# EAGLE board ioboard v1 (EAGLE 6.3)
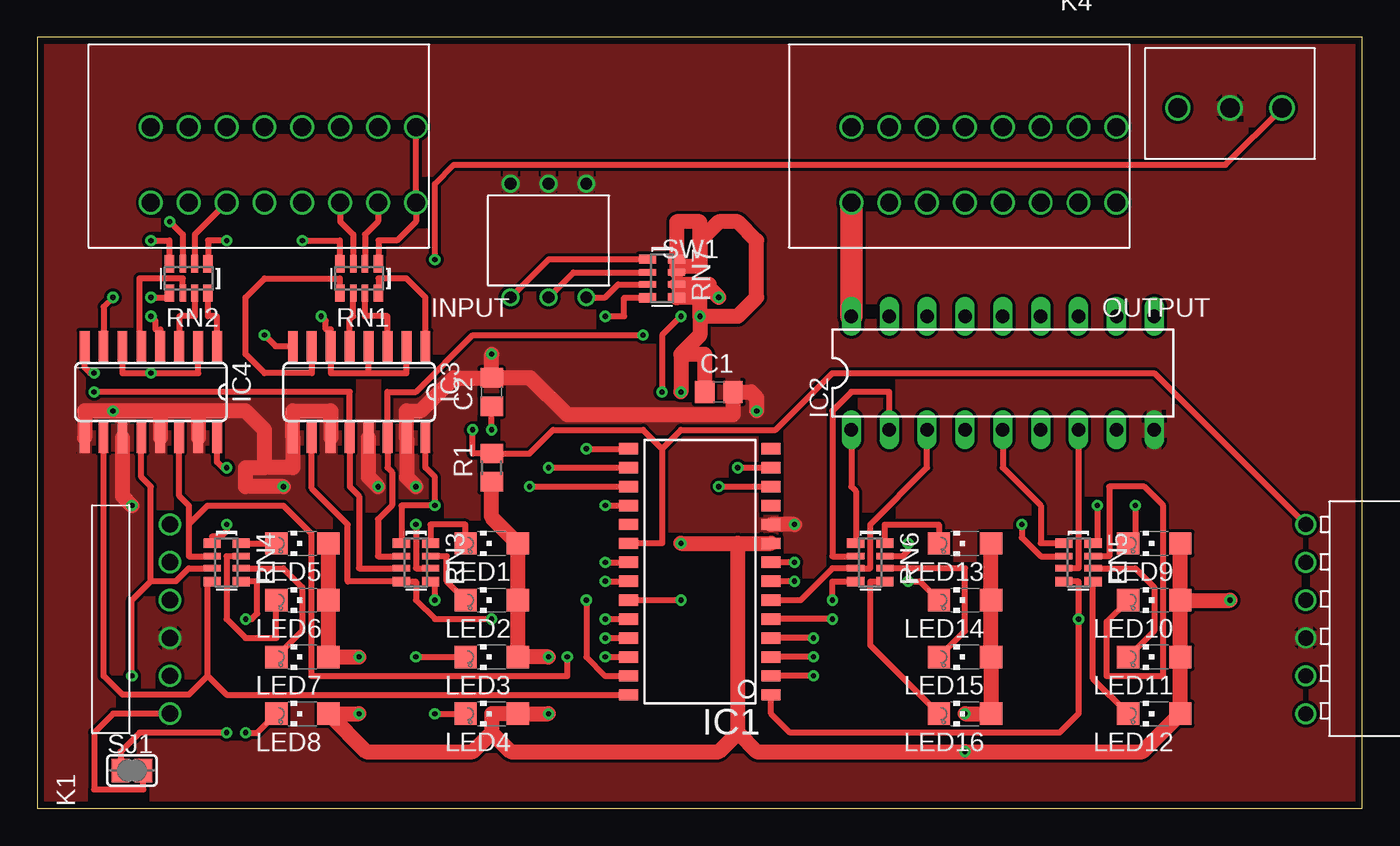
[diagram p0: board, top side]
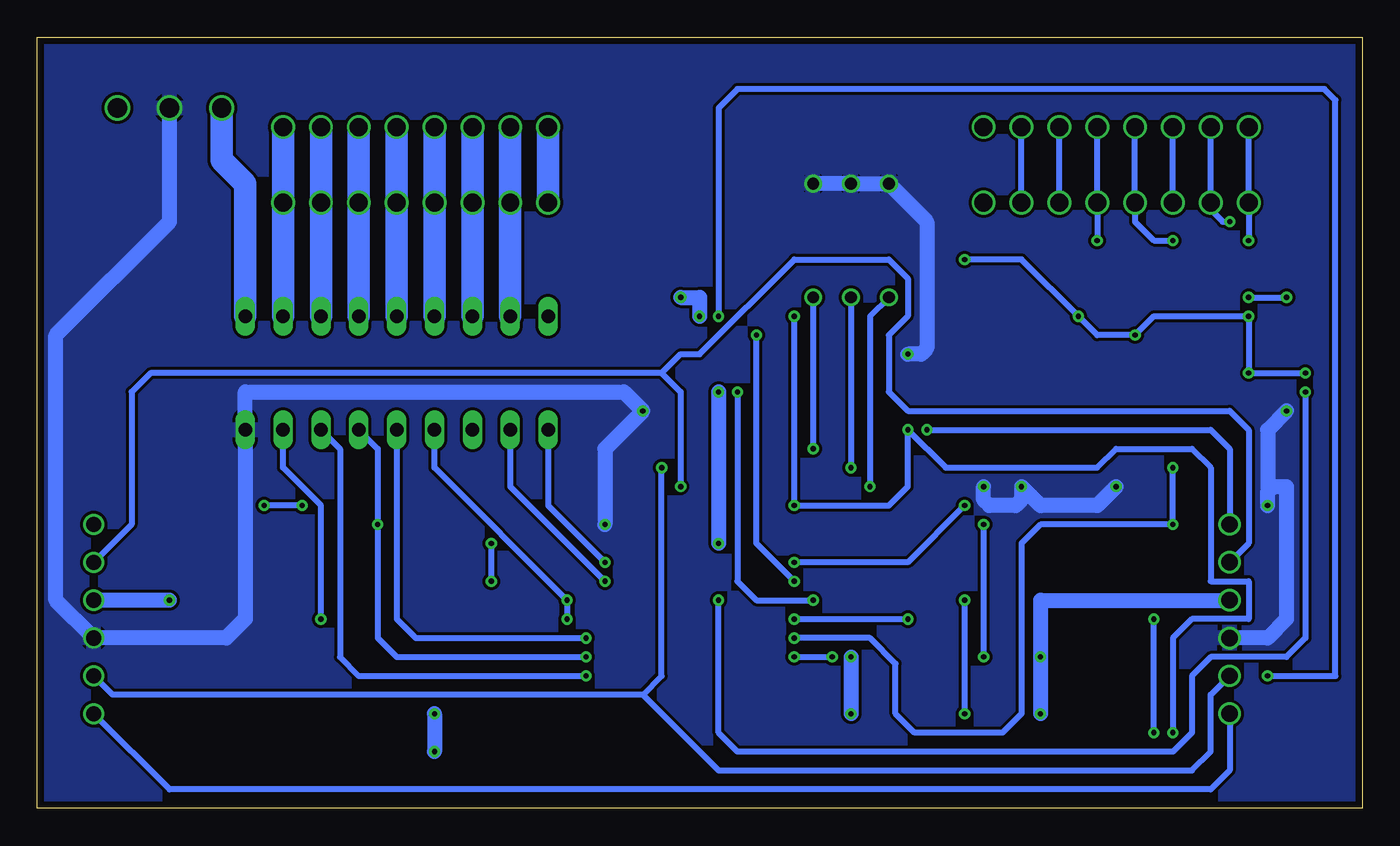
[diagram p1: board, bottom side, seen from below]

Size 88.88 x 51.74 mm. Coordinates in mm from the lower left corner, seen from the top.
Outline: 0,0 88.88,0 88.88,51.74 0,51.74 0,0
Copper layers (1*16): Top 0.018mm / dielectric 1.55mm / Bottom 0.018mm
Design rules "eC-STANDARD_pool-2-layer ": minimum track width 0.2mm, minimum drill 0.25mm, track to track 0.2mm, track to pad 0.2mm, pad to pad 0.2mm, via to via 0.2mm, smd to smd 0.15mm, copper to edge 0.45mm, drill to drill 0.3mm, minimum pad ring 0.2mm, minimum via ring 0.2mm, stop-mask expansion 0.1mm, vias tented up to drill 0mil, thermal gap 0.2mm
Net classes: 0 default: width 0.4 mm, drill 0.35 mm, clearance 0.2 mm; 1 power: width 1 mm, drill 0.35 mm, clearance 0.2 mm; 2 low_impedance: width 1.5 mm, drill 0.35 mm, clearance 0.2 mm

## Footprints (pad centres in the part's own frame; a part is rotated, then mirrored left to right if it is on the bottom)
C0805 = smd 1.3 x 1.5: 1 -0.95,0; 2 0.95,0
SO28W = smd 0.762 x 1.27: 1 -7.62,-4.78; 2 -6.35,-4.78; 3 -5.08,-4.78; 4 -3.81,-4.78; 5 -2.54,-4.78; 6 -1.27,-4.78; 7 0,-4.78; 8 1.27,-4.78; 9 2.54,-4.78; 10 3.81,-4.78; 11 5.08,-4.78; 12 6.35,-4.78; 13 7.62,-4.78; 14 8.89,-4.78; 15 8.89,4.78; 16 7.62,4.78; 17 6.35,4.78; 18 5.08,4.78; 19 3.81,4.78; 20 2.54,4.78; 21 1.27,4.78; 22 0,4.78; 23 -1.27,4.78; 24 -2.54,4.78; 25 -3.81,4.78; 26 -5.08,4.78; 27 -6.35,4.78; 28 -7.62,4.78
DIL18 = drill 0.9 long: 1 -10.16,-3.81; 2 -7.62,-3.81; 3 -5.08,-3.81; 4 -2.54,-3.81; 5 0,-3.81; 6 2.54,-3.81; 7 5.08,-3.81; 8 7.62,-3.81; 9 10.16,-3.81; 10 10.16,3.81; 11 7.62,3.81; 12 5.08,3.81; 13 2.54,3.81; 14 0,3.81; 15 -2.54,3.81; 16 -5.08,3.81; 17 -7.62,3.81; 18 -10.16,3.81
SO16 = smd 0.66 x 2.032: 1 -4.445,-3.073; 2 -3.175,-3.073; 3 -1.905,-3.073; 4 -0.635,-3.073; 5 0.635,-3.073; 6 1.905,-3.073; 7 3.175,-3.073; 8 4.445,-3.073; 9 4.445,3.073; 10 3.175,3.073; 11 1.905,3.073; 12 0.635,3.073; 13 -0.635,3.073; 14 -1.905,3.073; 15 -3.175,3.073; 16 -4.445,3.073
691402910008 = drill 1.2: 1 -10.16,0; 2 -7.62,0; 3 -5.08,0; 4 -2.54,0; 5 0,0; 6 2.54,0; 7 5.08,0; 8 7.62,0; 9 7.62,5.08; 10 5.08,5.08; 11 2.54,5.08; 12 0,5.08; 13 -2.54,5.08; 14 -5.08,5.08; 15 -7.62,5.08; 16 -10.16,5.08
61300611021 = drill 1.1: 1 6.35,0; 2 3.81,0; 3 1.27,0; 4 -1.27,0; 5 -3.81,0; 6 -6.35,0
613006143121 = drill 1.02: 1 0,0; 2 2.54,0; 3 5.08,0; 4 7.62,0; 5 10.16,0; 6 12.7,0
691214110003 = drill 1.3: 1 -3.5,0; 2 0,0; 3 3.5,0
CHIPLED_1206 = smd 1.5 x 1.5: A 0,-1.75; C 0,1.75
R0805 = smd 1.3 x 1.5: 1 -0.95,0; 2 0.95,0
RN8P-4R-CRA06S = smd 0.63 x 1.15: 1 -1.295,-0.975; 4 1.295,-0.975; 5 1.295,0.975; 8 -1.295,0.975 | smd 0.44 x 1.15: 2 -0.4,-0.975; 3 0.4,-0.975; 6 0.4,0.975; 7 -0.4,0.975
SJ = smd 1.168 x 1.6: 1 -0.762,0; 2 0.762,0
418127270903 = drill 0.8: 1 0,-3.81; 2 2.54,-3.81; 3 5.08,-3.81; 4 5.08,3.81; 5 2.54,3.81; 6 0,3.81

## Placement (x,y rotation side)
C1  [C0805]  45.72,27.94 0 top
C2  [C0805]  30.48,27.94 90 top
IC1  MCP23017SO  [SO28W]  44.45,15.24 90 top
IC2  [DIL18]  64.77,29.21 0 top
IC3  ACPL-244  [SO16]  21.59,27.94 180 top
IC4  ACPL-244  [SO16]  7.62,27.94 180 top
INPUT  691402910008  [691402910008]  15.24,45.72 180 top
K1  61300611021  [61300611021]  8.89,12.7 90 top
K2  613006143121  [613006143121]  85.09,19.05 270 top
K4  691214110003  [691214110003]  80.01,46.99 0 top
LED1  [CHIPLED_1206]  30.48,17.78 90 top
LED2  [CHIPLED_1206]  30.48,13.97 90 top
LED3  [CHIPLED_1206]  30.48,10.16 90 top
LED4  [CHIPLED_1206]  30.48,6.35 90 top
LED5  [CHIPLED_1206]  17.78,17.78 90 top
LED6  [CHIPLED_1206]  17.78,13.97 90 top
LED7  [CHIPLED_1206]  17.78,10.16 90 top
LED8  [CHIPLED_1206]  17.78,6.35 90 top
LED9  [CHIPLED_1206]  74.93,17.78 90 top
LED10  [CHIPLED_1206]  74.93,13.97 90 top
LED11  [CHIPLED_1206]  74.93,10.16 90 top
LED12  [CHIPLED_1206]  74.93,6.35 90 top
LED13  [CHIPLED_1206]  62.23,17.78 90 top
LED14  [CHIPLED_1206]  62.23,13.97 90 top
LED15  [CHIPLED_1206]  62.23,10.16 90 top
LED16  [CHIPLED_1206]  62.23,6.35 90 top
OUTPUT  691402910008  [691402910008]  62.23,45.72 180 top
R1  [R0805]  30.48,22.86 90 top
RN1  [RN8P-4R-CRA06S]  21.59,35.56 180 top
RN2  [RN8P-4R-CRA06S]  10.16,35.56 180 top
RN3  [RN8P-4R-CRA06S]  25.4,16.51 270 top
RN4  [RN8P-4R-CRA06S]  12.7,16.51 270 top
RN5  [RN8P-4R-CRA06S]  69.85,16.51 270 top
RN6  [RN8P-4R-CRA06S]  55.88,16.51 270 top
RN7  [RN8P-4R-CRA06S]  41.91,35.56 270 top
SJ1  [SJ]  6.35,2.54 0 top
SW1  418127270903  [418127270903]  36.83,38.1 180 top

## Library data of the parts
C1 C2 = rcl; MF: AVX; MPN: 08051A100JAT2A; OC_FARNELL: 499158
IC1 = adafruit; MF: MICROCHIP; MPN: MCP23017-E/SO; OC_FARNELL: 1332087
IC2 = ic; MF: TOSHIBA; MPN: ULN2803APG; OC_FARNELL: 1047761
IC3 IC4 = ic; MF: AVAGO TECHNOLOGIES; MPN: ACPL-244-500E; OC_FARNELL: 1634755
INPUT OUTPUT = Wuerth_Elektronik_eiCan_14_Terminal_Blocks_WR-TBL_2_0; OC_FARNELL: unknown
K1 K2 = Wuerth_Elektronik_eiCan_01_Pin__Socked_Headers_v1_3; OC_FARNELL: unknown
K4 = Wuerth_Elektronik_eiCan_14_Terminal_Blocks_WR-TBL_2_0; MF: WURTH ELEKTRONIK; MPN: 691214110003; OC_FARNELL: 1841251
LED1-LED16 = led; OC_FARNELL: unknown
R1 = rcl; OC_FARNELL: unknown
RN1-RN7 = dp_devices; OC_FARNELL: unknown
SJ1 = jumper; OC_FARNELL: unknown
SW1 = Eagle_Wuerth_Elektronik_Switch_Power_Elements; OC_FARNELL: unknown

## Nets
!RST: C2.1 IC1.18 RN7.4 SJ1.1
ADDR0: IC1.15 RN7.3 SW1.6
ADDR1: IC1.16 RN7.2 SW1.5
ADDR2: IC1.17 RN7.1 SW1.4
AGND: IC3.2 IC3.4 IC3.6 IC3.8 IC4.2 IC4.4 IC4.6 IC4.8 K4.3
GND [power]: C1.2 C2.2 IC1.10 IC2.9 IC3.9 IC3.11 IC3.13 IC3.15 IC4.9 IC4.11 IC4.13 IC4.15 K1.4 K2.4 K4.2 SW1.1 SW1.2 SW1.3
IN0: INPUT.1 INPUT.16 RN1.1
IN1: INPUT.2 INPUT.15 RN1.2
IN2: INPUT.3 INPUT.14 RN1.3
IN3: INPUT.4 INPUT.13 RN1.4
IN4: INPUT.5 INPUT.12 RN2.1
IN5: INPUT.6 INPUT.11 RN2.2
IN6: INPUT.7 INPUT.10 RN2.3
IN7: INPUT.8 INPUT.9 RN2.4
IN_L0: IC1.21 IC3.16 RN3.1
IN_L1: IC1.22 IC3.14 RN3.2
IN_L2: IC1.23 IC3.12 RN3.3
IN_L3: IC1.24 IC3.10 RN3.4
IN_L4: IC1.25 IC4.16 RN4.1
IN_L5: IC1.26 IC4.14 RN4.2
IN_L6: IC1.27 IC4.12 RN4.3
IN_L7: IC1.28 IC4.10 RN4.4
INT: IC1.20 K1.1 K2.1 R1.2
N$9: IC3.1 RN1.8
N$10: IC3.3 RN1.7
N$11: IC3.5 RN1.6
N$12: IC3.7 RN1.5
N$13: IC4.1 RN2.8
N$14: IC4.3 RN2.7
N$15: IC4.5 RN2.6
N$16: IC4.7 RN2.5
N$17: LED1.C RN3.8
N$18: LED2.C RN3.7
N$25: LED9.C RN5.8
N$26: LED10.C RN5.7
N$27: LED11.C RN5.6
N$28: LED12.C RN5.5
N$29: LED3.C RN3.6
N$30: LED4.C RN3.5
N$31: LED13.C RN6.8
N$32: LED14.C RN6.7
N$33: LED15.C RN6.6
N$34: LED16.C RN6.5
N$36: LED5.C RN4.8
N$37: LED6.C RN4.7
N$38: LED7.C RN4.6
N$39: LED8.C RN4.5
OUT0 [low_impedance]: IC2.11 OUTPUT.1 OUTPUT.16
OUT1 [low_impedance]: IC2.12 OUTPUT.2 OUTPUT.15
OUT2 [low_impedance]: IC2.13 OUTPUT.3 OUTPUT.14
OUT3 [low_impedance]: IC2.14 OUTPUT.4 OUTPUT.13
OUT4 [low_impedance]: IC2.15 OUTPUT.5 OUTPUT.12
OUT5 [low_impedance]: IC2.16 OUTPUT.6 OUTPUT.11
OUT6 [low_impedance]: IC2.17 OUTPUT.7 OUTPUT.10
OUT7 [low_impedance]: IC2.18 OUTPUT.8 OUTPUT.9
OUT_L0: IC1.1 IC2.8 RN5.4
OUT_L1: IC1.2 IC2.7 RN5.3
OUT_L2: IC1.3 IC2.6 RN5.2
OUT_L3: IC1.4 IC2.5 RN5.1
OUT_L4: IC1.5 IC2.4 RN6.4
OUT_L5: IC1.6 IC2.3 RN6.3
OUT_L6: IC1.7 IC2.2 RN6.2
OUT_L7: IC1.8 IC2.1 RN6.1
RST_EXT: K1.6 K2.6 SJ1.2
SCL: IC1.12 K1.2 K2.2
SDA: IC1.13 K1.5 K2.5
V+ [low_impedance]: IC2.10 K4.1
VDD [power]: C1.1 IC1.9 K1.3 K2.3 LED1.A LED2.A LED3.A LED4.A LED5.A LED6.A LED7.A LED8.A LED9.A LED10.A LED11.A LED12.A LED13.A LED14.A LED15.A LED16.A R1.1 RN7.5 RN7.6 RN7.7 RN7.8

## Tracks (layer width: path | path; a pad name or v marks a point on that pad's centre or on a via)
!RST  (via drill 0.35 pad 0.75)
  Top 0.4: v12.7,5.08 6.86,5.08 5.59,3.81 SJ1.1 | v38.1,33.02 39.37,33.02 39.37,34.27 RN7.4 | v30.48,25.4 C2.1 | v38.1,20.32 IC1.18
  Bottom 0.4: v12.7,5.08 12.7,11.43 11.43,12.7 7.62,12.7 7.62,15.24 10.16,15.24 10.16,22.86 11.43,24.13 16.51,24.13 17.78,22.86 27.94,22.86 v30.48,25.4 30.48,21.59 31.75,20.32 v38.1,20.32 v38.1,33.02
ADDR0  (via drill 0.35 pad 0.75)
  Top 0.4: SW1.6 38.1,34.29 38.97,35.16 RN7.3 | v36.83,24.13 IC1.15
  Bottom 0.4: SW1.6 v36.83,24.13
ADDR1  (via drill 0.35 pad 0.75)
  Top 0.4: SW1.5 35.96,35.96 RN7.2 | v34.29,22.86 IC1.16
  Bottom 0.4: SW1.5 v34.29,22.86
ADDR2  (via drill 0.35 pad 0.75)
  Top 0.4: SW1.4 34.31,36.85 RN7.1 | v33.02,21.59 IC1.17
  Bottom 0.4: SW1.4 33.02,33.02 v33.02,21.59
AGND  (via drill 0.35 pad 0.75)
  Top 0.4: IC3.2 24.77,29.21 22.23,29.21 | 22.23,29.21 19.68,29.21 IC3.6 19.68,32.14 19.34,32.14 19.34,32.73 v19.05,33.02 | IC4.2 10.79,29.21 v7.62,29.21 5.71,29.21 IC4.6 | 22.23,29.21 IC3.4 | v3.81,29.21 3.55,29.21 3.17,29.59 IC4.8 | v26.67,36.83 26.67,41.91 27.94,43.18 79.7,43.18 K4.3 | v7.62,33.02 7.92,32.73 7.92,32.14 8.26,32.14 IC4.4 | v15.24,31.75 15.98,31.01 IC3.8
  Bottom 0.4: v3.81,29.21 v7.62,29.21 v7.62,33.02 13.97,33.02 v15.24,31.75 17.78,31.75 v19.05,33.02 22.86,36.83 v26.67,36.83
GND  (via drill 0.35 pad 0.75)
  Top 1: 15.24,22.86 15.24,25.4 13.97,26.67 10.79,26.67 | 10.79,26.67 8.26,26.67 | 10.79,26.67 IC4.15 | C2.2 27.94,28.89 25.72,26.67 24.77,26.67 IC3.15 24.77,22.23 v25.4,21.59 | C2.2 33.06,28.89 35.56,26.39 46.67,26.39 C1.2 47.88,27.94 48.26,27.57 v48.26,26.67 | 15.24,22.86 17.14,22.86 IC3.9 17.14,26.67 19.68,26.67 IC3.11 | v16.51,21.59 13.97,21.59 13.97,22.86 15.24,22.86 | 8.26,26.67 v5.08,26.67 3.17,26.67 IC4.9 | 8.26,26.67 IC4.13 | C2.2 v30.48,30.48 | v50.8,19.05 IC1.10 | v22.86,21.59 22.23,22.23 IC3.13 | v6.35,20.32 5.71,20.95 IC4.11
  Bottom 1: 6.35,21.21 5.97,21.59 5.08,21.59 5.08,12.7 6.35,11.43 K1.4 | v5.08,26.67 6.35,25.4 6.35,21.21 | K4.2 80.01,39.37 87.63,31.75 87.63,13.97 K2.4 76.2,11.43 74.93,12.7 IC2.9 74.93,27.94 49.53,27.94 v48.26,26.67 50.8,24.13 v50.8,19.05 | v6.35,20.32 6.35,21.21 | v16.51,21.59 17.78,20.32 21.59,20.32 v22.86,21.59 22.86,20.7 23.23,20.32 25.02,20.32 25.4,20.7 v25.4,21.59 | SW1.1 SW1.2 SW1.3 29.21,39.37 29.21,30.86 29.59,30.48 v30.48,30.48
  pour Top (isolate 0.2): 0,0 0,52.07 88.9,52.07 88.9,0
  pour Bottom (isolate 0.2): 0,0 0,52.07 88.9,52.07 88.9,0
IN0
  Top 0.4: RN1.1 22.89,38.1 24.13,38.1 25.4,39.37 INPUT.16 INPUT.1
IN1
  Top 0.4: INPUT.15 22.86,39.37 21.99,38.5 RN1.2
  Bottom 0.4: INPUT.15 INPUT.2
IN2
  Top 0.4: INPUT.14 20.32,39.37 21.19,38.5 RN1.3
  Bottom 0.4: INPUT.14 INPUT.3
IN3  (via drill 0.35 pad 0.75)
  Top 0.4: v17.78,38.1 20.3,38.1 RN1.4
  Bottom 0.4: INPUT.4 INPUT.13 v17.78,38.1
IN4  (via drill 0.35 pad 0.75)
  Top 0.4: v12.7,38.1 11.46,38.1 RN2.1
  Bottom 0.4: v12.7,38.1 13.97,38.1 15.24,39.37 INPUT.12 INPUT.5
IN5
  Top 0.4: INPUT.11 10.56,38.5 RN2.2
  Bottom 0.4: INPUT.11 INPUT.6
IN6  (via drill 0.35 pad 0.75)
  Top 0.4: v8.89,39.37 9.76,38.5 RN2.3
  Bottom 0.4: v8.89,39.37 9.36,39.37 10.16,40.17 INPUT.10 INPUT.7
IN7  (via drill 0.35 pad 0.75)
  Top 0.4: v7.62,38.1 8.87,38.1 RN2.4
  Bottom 0.4: INPUT.8 INPUT.9 v7.62,38.1
IN_L0  (via drill 0.35 pad 0.75)
  Top 0.4: RN3.1 24.43,20.32 v26.67,20.32 26.67,22.23 26.04,22.86 IC3.16 | v38.1,16.51 IC1.21
  Bottom 0.4: v26.67,20.32 30.48,16.51 v38.1,16.51
IN_L1  (via drill 0.35 pad 0.75)
  Top 0.4: RN3.2 22.86,16.91 22.86,19.39 23.79,20.32 23.79,22.56 23.5,22.86 IC3.14 23.5,27.94 25.4,27.94 29.21,31.75 v40.64,31.75 | v38.1,15.24 IC1.22
  Bottom 0.4: v38.1,15.24 40.64,17.78 v40.64,31.75
IN_L2  (via drill 0.35 pad 0.75)
  Top 0.4: RN3.3 21.59,16.11 21.59,20.95 20.95,21.59 IC3.12 20.95,27.94 v3.81,27.94 | v43.18,13.97 IC1.23
  Bottom 0.4: v3.81,27.94 3.81,11.43 5.08,10.16 10.16,10.16 11.43,8.89 11.43,5.08 12.7,3.81 41.91,3.81 43.18,5.08 v43.18,13.97
IN_L3  (via drill 0.35 pad 0.75)
  Top 0.4: IC3.10 18.41,21.47 20.84,19.05 20.84,15.21 RN3.4 25.4,15.21 25.4,13.97 26.67,12.7 v30.48,12.7 | v38.1,12.7 IC1.24
  Bottom 0.4: v38.1,12.7 v30.48,12.7
IN_L4  (via drill 0.35 pad 0.75)
  Top 0.4: v12.7,22.86 12.44,22.86 12.06,23.23 IC4.16 | v38.1,11.43 IC1.25 | v12.7,19.05 12.7,18.61 12.32,18.24 11.72,18.24 RN4.1
  Bottom 0.4: v12.7,22.86 v12.7,19.05 21.59,19.05 22.86,17.78 22.86,6.35 24.13,5.08 30.03,5.08 31.3,6.35 31.3,9.71 33.02,11.43 v38.1,11.43
IN_L5  (via drill 0.35 pad 0.75)
  Top 0.4: 10.16,19.05 10.16,20.32 9.53,20.95 IC4.14 | 10.16,19.05 10.16,16.91 RN4.2 | 10.16,19.05 11.43,20.32 16.51,20.32 18.38,18.45 18.38,8.89 35.56,8.89 v35.56,10.16 | v38.1,10.16 IC1.26
  Bottom 0.4: v38.1,10.16 v35.56,10.16
IN_L6  (via drill 0.35 pad 0.75)
  Top 0.4: 7.62,15.24 7.62,21.59 6.99,22.23 IC4.12 | v6.35,8.89 6.35,13.97 7.62,15.24 | 7.62,15.24 9.29,15.24 10.16,16.11 RN4.3 | v36.83,13.97 36.83,10.16 38.1,8.89 IC1.27 | v43.18,33.02 41.91,31.75 v41.91,27.94
  Bottom 0.4: v41.91,27.94 41.91,15.24 40.64,13.97 v36.83,13.97 | v6.35,8.89 1.8,8.89 1.8,47.52 2.54,48.26 41.91,48.26 43.18,46.99 v43.18,33.02
IN_L7
  Top 0.4: 11.43,8.89 10.16,7.62 5.71,7.62 4.45,8.89 IC4.10 | 11.43,8.89 11.43,15.21 RN4.4 | 11.43,8.89 12.7,7.62 IC1.28
INT  (via drill 0.35 pad 0.75)
  Top 0.4: 41.91,24.13 40.64,25.4 34.61,25.4 33.02,23.81 R1.2 29.21,23.81 v29.21,25.4 | 41.91,24.13 41.91,17.78 IC1.20 | 41.91,24.13 43.18,25.4 49.53,25.4 53.34,29.21 74.93,29.21 K2.1
  Bottom 0.4: v29.21,25.4 10.16,25.4 8.89,24.13 K1.1
N$9
  Top 0.4: IC3.1 26.04,34.29 24.77,35.56 22.89,35.56 RN1.8
N$10
  Top 0.4: IC3.3 23.5,33.02 21.99,33.02 RN1.7
N$11
  Top 0.4: IC3.5 20.95,32.78 21.19,33.02 RN1.6
N$12
  Top 0.4: IC3.7 18.41,29.21 15.24,29.21 13.97,30.48 13.97,34.29 15.24,35.56 20.3,35.56 RN1.5
N$13
  Top 0.4: IC4.1 12.06,33.02 11.46,33.02 RN2.8
N$14
  Top 0.4: RN2.7 10.56,33.02 9.53,33.02 IC4.3
N$15
  Top 0.4: RN2.6 9.76,35.56 6.84,35.56 6.84,31.01 IC4.5
N$16  (via drill 0.35 pad 0.75)
  Top 0.4: v5.08,34.29 4.45,33.66 IC4.7 | v7.62,34.29 8.87,34.29 RN2.5
  Bottom 0.4: v7.62,34.29 v5.08,34.29
N$17
  Top 0.4: LED1.C 28.73,19.05 26.38,19.05 RN3.8
N$18
  Top 0.4: LED2.C 27.46,15.23 27.46,16.91 RN3.7
N$25  (via drill 0.35 pad 0.75)
  Top 0.4: v73.66,20.32 73.66,18.26 LED9.C | v71.12,20.32 71.12,17.8 RN5.8
  Bottom 0.4: v71.12,20.32 v73.66,20.32
N$26
  Top 0.4: LED10.C 71.73,12.52 71.73,8.89 75.53,8.89 75.53,20.32 74.26,21.59 71.92,21.59 71.92,16.91 RN5.7
N$27
  Top 0.4: RN5.6 73.66,16.11 74.93,14.84 74.93,11.91 LED11.C
N$28
  Top 0.4: LED12.C 70.83,8.71 RN5.5
N$29  (via drill 0.35 pad 0.75)
  Top 0.4: v25.4,10.16 LED3.C | v25.4,19.05 25.4,16.11 RN3.6
  Bottom 0.4: v25.4,19.05 v25.4,10.16
N$30  (via drill 0.35 pad 0.75)
  Top 0.4: v26.67,6.35 LED4.C | v26.67,13.97 26.67,15.21 RN3.5
  Bottom 0.4: v26.67,13.97 v26.67,6.35
N$31
  Top 0.4: RN6.8 56.85,19.05 60.48,19.05 LED13.C
N$32  (via drill 0.35 pad 0.75)
  Top 0.4: v58.42,17.78 58.42,17.29 58.05,16.91 RN6.7 | v58.42,15.24 59.21,15.24 LED14.C
  Bottom 0.4: v58.42,15.24 v58.42,17.78
N$33
  Top 0.4: LED15.C 62.23,11.91 62.23,16.11 RN6.6
N$34
  Top 0.4: LED16.C 55.88,10.95 55.88,15.21 RN6.5
N$36
  Top 0.4: RN4.8 13.97,17.8 13.99,17.78 LED5.C
N$37
  Top 0.4: RN4.7 12.7,16.91 12.7,12.7 13.97,11.43 16.03,11.43 LED6.C
N$38
  Top 0.4: RN4.6 16.51,16.11 17.78,14.84 17.78,11.91 LED7.C
N$39  (via drill 0.35 pad 0.75)
  Top 0.4: v13.97,12.7 14.39,12.7 14.77,13.07 14.77,15.21 RN4.5 | v13.97,5.08 14.76,5.08 LED8.C
  Bottom 0.4: v13.97,5.08 v13.97,12.7
OUT0
  Bottom 1.5: IC2.11 OUTPUT.16 OUTPUT.1
OUT1
  Bottom 1.5: IC2.12 OUTPUT.15 OUTPUT.2
OUT2
  Bottom 1.5: IC2.13 OUTPUT.14 OUTPUT.3
OUT3
  Bottom 1.5: IC2.14 OUTPUT.13 OUTPUT.4
OUT4
  Bottom 1.5: IC2.15 OUTPUT.12 OUTPUT.5
OUT5
  Bottom 1.5: IC2.16 OUTPUT.11 OUTPUT.6
OUT6
  Bottom 1.5: IC2.17 OUTPUT.10 OUTPUT.7
OUT7
  Top 1.5: OUTPUT.9 IC2.18
  Bottom 1.5: OUTPUT.9 OUTPUT.8
OUT_L0  (via drill 0.35 pad 0.75)
  Top 0.4: IC1.1 49.23,6.35 50.5,5.08 68.58,5.08 69.85,6.35 v69.85,12.7 69.85,15.21 RN5.4
  Bottom 0.4: v69.85,12.7 69.85,20.32 72.39,22.86 IC2.8
OUT_L1  (via drill 0.35 pad 0.75)
  Top 0.4: IC2.7 69.85,16.11 RN5.3 | v52.07,8.89 IC1.2
  Bottom 0.4: IC2.7 68.58,24.13 68.58,10.16 67.31,8.89 v52.07,8.89
OUT_L2  (via drill 0.35 pad 0.75)
  Top 0.4: v52.07,10.16 IC1.3 | v66.04,19.05 66.04,18.18 67.31,16.91 RN5.2
  Bottom 0.4: IC2.6 66.04,24.13 v66.04,19.05 66.04,11.43 64.77,10.16 v52.07,10.16
OUT_L3  (via drill 0.35 pad 0.75)
  Top 0.4: IC2.5 64.77,22.86 67.31,20.32 67.31,17.8 RN5.1 | v52.07,11.43 IC1.4
  Bottom 0.4: IC2.5 64.77,12.7 63.5,11.43 v52.07,11.43
OUT_L4  (via drill 0.35 pad 0.75)
  Top 0.4: v53.34,12.7 IC1.5 | v53.34,13.97 53.34,15.21 RN6.4
  Bottom 0.4: IC2.4 62.23,22.86 v53.34,13.97 v53.34,12.7
OUT_L5
  Top 0.4: IC2.3 59.69,22.86 55.88,19.05 55.88,16.11 RN6.3 53.34,16.11 51.2,13.97 IC1.6
OUT_L6  (via drill 0.35 pad 0.75)
  Top 0.4: IC2.2 57.15,27.94 54.61,27.94 53.34,26.67 53.34,16.91 RN6.2 | v50.8,15.24 IC1.7
  Bottom 0.4: IC2.2 57.15,21.59 v50.8,15.24
OUT_L7  (via drill 0.35 pad 0.75)
  Top 0.4: IC2.1 54.61,21.59 54.91,21.3 RN6.1 | v50.8,16.51 IC1.8
  Bottom 0.4: IC2.1 54.61,20.32 v50.8,16.51
RST_EXT
  Top 0.4: K1.6 5.08,6.35 3.81,5.08 3.81,1.27 7.11,1.27 SJ1.2
  Bottom 0.4: K1.6 8.89,2.54 10.16,1.27 80.01,1.27 K2.6
SCL  (via drill 0.35 pad 0.75)
  Top 0.4: v45.72,21.59 IC1.12
  Bottom 0.4: 46.99,29.21 81.28,29.21 82.55,27.94 82.55,19.05 K2.2 | 46.99,29.21 45.72,30.48 44.45,30.48 38.1,36.83 31.75,36.83 30.48,35.56 30.48,33.02 31.75,31.75 31.75,27.94 30.48,26.67 8.89,26.67 7.62,25.4 7.62,17.78 K1.2 | 46.99,29.21 45.72,27.94 v45.72,21.59
SDA  (via drill 0.35 pad 0.75)
  Top 0.4: v46.99,22.86 IC1.13
  Bottom 0.4: 48.26,7.62 43.18,2.54 11.43,2.54 10.16,3.81 10.16,7.62 K1.5 | 48.26,7.62 83.82,7.62 K2.5 | 48.26,7.62 46.99,8.89 v46.99,22.86
V+
  Bottom 1.5: K4.1 76.51,43.49 74.93,41.91 IC2.10
VDD  (via drill 0.35 pad 0.75)
  Top 1: v34.29,10.16 LED3.A LED2.A LED1.A 30.48,19.53 R1.1 | 46.99,5.08 46.99,17.78 | v43.18,17.78 46.99,17.78 | v62.23,6.35 LED16.A LED15.A LED14.A LED13.A | 30.48,5.08 29.21,3.81 22.07,3.81 LED8.A v21.59,6.35 | 30.48,5.08 30.48,6.35 LED4.A v34.29,6.35 | 44.45,38.1 44.45,39.37 42.88,39.37 RN7.8 | 43.18,30.48 44.77,30.48 C1.1 | 46.99,17.78 IC1.9 | v44.45,33.02 46.99,33.02 48.26,34.29 48.26,38.1 46.99,39.37 45.72,39.37 44.45,38.1 | 30.48,5.08 31.75,3.81 45.72,3.81 46.99,5.08 | LED10.A LED11.A LED12.A 74.14,3.81 v62.23,3.81 48.26,3.81 46.99,5.08 | LED10.A LED9.A | LED5.A LED6.A LED7.A v21.59,10.16 | LED10.A v80.01,13.97 | v44.45,33.02 44.45,31.75 43.18,30.48 | 44.45,38.1 44.45,36.36 42.88,36.36 RN7.7 | 43.18,30.48 v43.18,27.94 | v44.45,33.02 44.45,34.27 RN7.5 | v45.72,34.29 45.09,34.92 45.09,35.16 RN7.6
  Bottom 1: K1.3 21.59,13.97 v21.59,10.16 v21.59,6.35 | v80.01,13.97 K2.3 | v34.29,10.16 v34.29,6.35 | v62.23,6.35 v62.23,3.81 | v43.18,27.94 v43.18,17.78 | v44.45,33.02 44.45,34.29 v45.72,34.29

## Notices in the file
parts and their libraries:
Wuerth_Elektronik_eiCan_01_Pin__Socked_H: Copyright: Würth Elektronik
